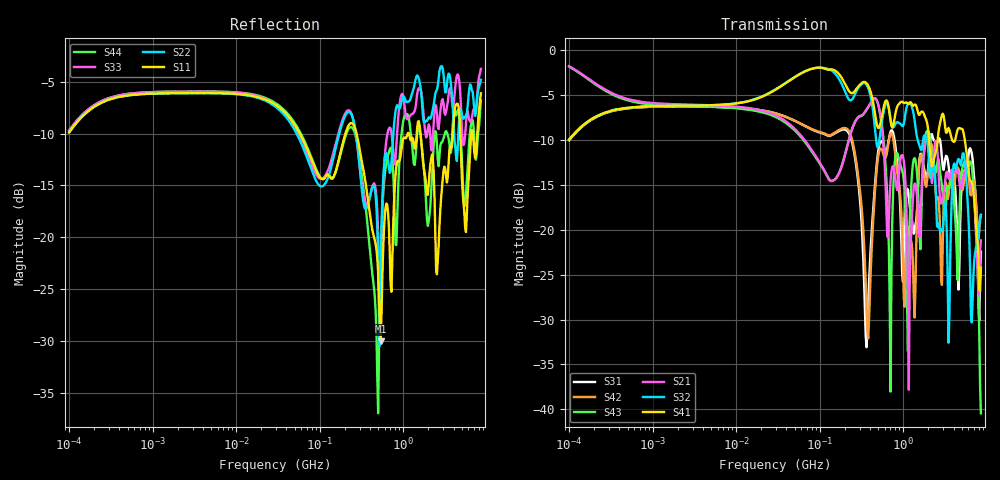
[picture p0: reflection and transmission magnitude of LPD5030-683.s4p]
# MHz S MA R 50
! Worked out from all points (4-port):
!   498 points, 100 kHz to 8.5 GHz, reference 50 ohm
!   strongest paths, dB at 100 kHz, 1.698 MHz, 29.49 MHz, 500.7 MHz, 8.5 GHz:
!     S41: -10.0, -6.2, -4.4, -8.7, -24.2
!     S32: -10.0, -6.2, -4.4, -10.8, -18.3
!     S21: -1.8, -6.0, -7.2, -6.0, -21.2
!     S43: -1.8, -6.2, -7.4, -6.0, -40.5
!     S42: -10.0, -6.3, -7.0, -11.9, -18.4
!     S31: -10.0, -6.3, -7.0, -11.3, -22.4
!   lowest |S11| = -30.0 dB at 536.2 MHz (marker M1), VSWR 1.06, Z = 48.8 + j2.86 ohm
!   |S11| at or under -10 dB: 276.4 MHz to 1.131 GHz (854.8 MHz wide, 121 % of centre); 1.61 GHz to 3.926 GHz (2.316 GHz wide, 83.7 % of centre); 4.818 GHz to 6.537 GHz (1.718 GHz wide, 30.3 % of centre)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
0.1  0.3211 47.7  0.815 -17.1  0.3153 -130.8  0.318 49.2
     0.815 -17.1  0.3198 47.8  0.3174 49.4  0.3153 -131.1
     0.3153 -130.8  0.3174 49.4  0.3269 47.7  0.811 -17.5
     0.318 49.2  0.3153 -131.1  0.811 -17.5  0.3271 47.7
205.4604  0.3216 -31.6  0.2709 134.7  0.3599 -2.4  0.6367 -46.5
          0.2709 134.7  0.3912 -24.5  0.5749 -52.4  0.3679 -3.5
          0.3599 -2.4  0.5749 -52.4  0.4003 -26.3  0.274 132.4
          0.6367 -46.5  0.3679 -3.5  0.274 132.4  0.311 -33.0
363.6528  0.1701 -107.2  0.4677 6.8  0.02216 -24.2  0.6549 -70.0
          0.4677 6.8  0.1376 -55.5  0.6416 -79.6  0.03741 -74.8
          0.02216 -24.2  0.6416 -79.6  0.144 -58.8  0.4651 4.7
          0.6549 -70.0  0.03741 -74.8  0.4651 4.7  0.1279 -109.6
536.1655  0.03145 111.5  0.4215 -93.1  0.3106 -27.9  0.3962 -78.5
          0.4215 -93.1  0.06477 14.9  0.3544 -80.5  0.2837 -36.0
          0.3106 -27.9  0.3544 -80.5  0.04744 -5.4  0.4265 -96.5
          0.3962 -78.5  0.2837 -36.0  0.4265 -96.5  0.08094 42.1
705.2109  0.05985 -74.3  0.1873 -73.2  0.3523 -86.2  0.4034 -112.6
          0.1873 -73.2  0.2081 -36.4  0.4141 -125.1  0.343 -95.0
          0.3523 -86.2  0.4141 -125.1  0.3352 -59.4  0.01253 32.7
          0.4034 -112.6  0.343 -95.0  0.01253 32.7  0.2701 -67.1
6462.473  0.3042 -83.5  0.1716 -119.4  0.2781 -137.4  0.1861 -159.3
          0.1716 -119.4  0.5389 -113.7  0.03329 160.4  0.1552 -122.9
          0.2781 -137.4  0.03329 160.4  0.3638 -103.6  0.2385 -126.5
          0.1861 -159.3  0.1552 -122.9  0.2385 -126.5  0.3474 -96.8
8500  0.495 -36.3  0.08727 28.8  0.07546 0.1  0.06162 -22.9
      0.08727 28.8  0.5755 -49.2  0.1211 79.2  0.1209 -7.8
      0.07546 0.1  0.1211 79.2  0.6493 -37.2  0.009494 -25.2
      0.06162 -22.9  0.1209 -7.8  0.009494 -25.2  0.458 -33.3
